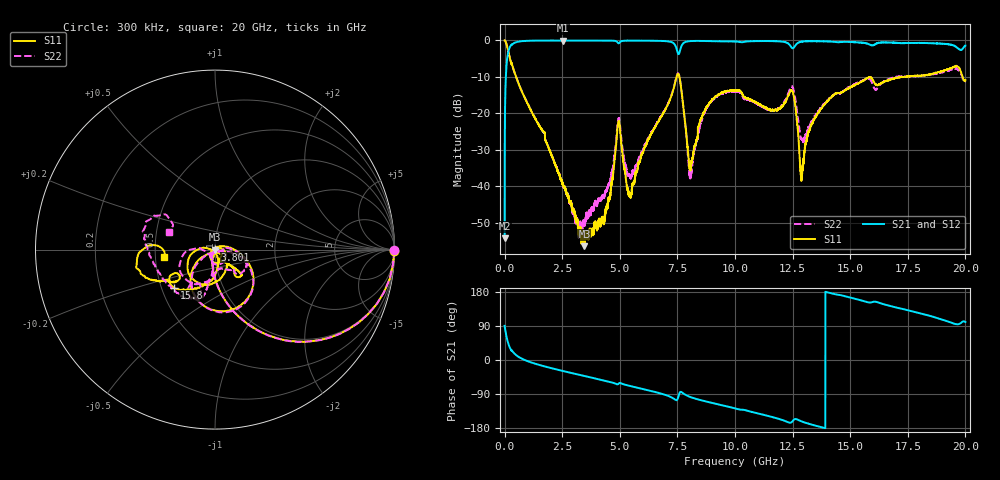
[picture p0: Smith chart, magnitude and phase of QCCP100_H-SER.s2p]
!{QCCP100}
!Johanson Technology Inc.
!www.johansontechnology.com
!Test Board Conditions:
!Substrate Type  RO4350B
!Substrate Thickness  20 mil
!Substrate Dk  3.66
!TL Type: GCPW
!TL Trace Width  36 mil
!TL Gap  12 mil
!Electrode orientation  Horizontal
!DUT TOPOLOGY	SERIES
!Mounting Pad LxW  26x36 mil
! Created Sat Jan  9 18:32:08 2021
# hz S ma R 50
! 2 Port Network Data from SP1.SP block
! freq  magS11  angS11  magS21  angS21  magS12  angS12  magS22  angS22
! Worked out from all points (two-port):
!   20001 points, 300 kHz to 20 GHz, reference 50 ohm
!   highest |S21| = -0.02 dB at 2.53 GHz (marker M1); lowest = -54.2 dB at 300 kHz (marker M2)
!   |S21| within 3 dB of the highest: 162.7 MHz to 7.498 GHz (7.336 GHz wide, 192 % of centre); 7.603 GHz to end of sweep
!   lowest |S11| = -56.4 dB at 3.465 GHz (marker M3), VSWR 1.00, Z = 49.9 - j0.048 ohm
!   |S11| at or under -10 dB: 496.9 MHz to 7.463 GHz (6.966 GHz wide, 175 % of centre); 7.588 GHz to 17.21 GHz (9.617 GHz wide, 77.6 % of centre); 19.87 GHz to end of sweep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
!   |S22| runs from -54.2 to 0.0 dB; largest |S21 - S12| = 0.018
!   S11 on the Smith chart (normalised r, x): 300 kHz: open; 3.801 GHz: 1.00, +0.00; 15.8 GHz: 0.58, -0.28; 20 GHz: 0.56, -0.05
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300000  0.9995 -0.4  0.001944 90.1  0.001894 89.9  0.9999 -0.3
1.063e8  0.8343 -34.5  0.5474 55.3  0.5485 55.2  0.8345 -34.5
2.403e8  0.5534 -58.7  0.8276 30.8  0.8287 30.8  0.5544 -58.8
2.5303e9  0.01036 -93.8  0.998 -29.0  0.9964 -29.0  0.01054 -142.2
3.3343e9  0.002096 -140.7  0.996 -40.4  0.9956 -40.4  0.002218 -88.4
3.4653e9  0.001514 -161.5  0.9962 -42.2  0.9966 -42.2  0.00308 -69.3
3.8013e9  0.002338 150.4  0.9963 -46.9  0.9963 -46.9  0.005193 -53.2
4.3843e9  0.004806 75.8  0.9959 -55.1  0.9951 -55.1  0.00868 -29.5
4.9393e9  0.07748 -52.5  0.9159 -63.0  0.915 -63.0  0.08473 -57.3
5.4303e9  0.007658 120.9  0.9935 -68.3  0.9935 -68.3  0.01387 -74.2
6.6673e9  0.0771 9.3  0.9886 -86.6  0.9877 -86.6  0.07832 -9.0
7.5483e9  0.3448 -85.2  0.6484 -95.6  0.6493 -95.6  0.3515 -83.9
8.0713e9  0.01803 -79.8  0.9804 -97.9  0.9804 -97.8  0.01349 -61.3
8.8173e9  0.1274 -45.0  0.9821 -110.6  0.9809 -110.6  0.1233 -5.7
1.00003e10  0.2053 -44.5  0.9679 -127.6  0.967 -127.6  0.1977 -34.9
1.16303e10  0.1119 -48.8  0.9798 -150.8  0.9793 -150.7  0.1112 -75.7
1.24673e10  0.2066 -124.0  0.7926 -163.6  0.7964 -163.6  0.2324 -137.6
1.28953e10  0.01306 -117.4  0.9643 -162.0  0.9653 -162.1  0.04509 -152.1
1.33343e10  0.07168 -75.1  0.9778 -170.6  0.9801 -170.6  0.07831 -98.6
1.57963e10  0.3121 -136.8  0.8938 152.0  0.8972 151.8  0.3004 -115.2
1.66673e10  0.2844 -141.1  0.9348 143.6  0.9307 143.5  0.2938 -114.8
2e10  0.2847 -171.0  0.8526 100.3  0.8464 100.2  0.2768 159.3
